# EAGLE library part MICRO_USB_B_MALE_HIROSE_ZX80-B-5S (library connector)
CONN PLUG MCR USB B PCB VERT
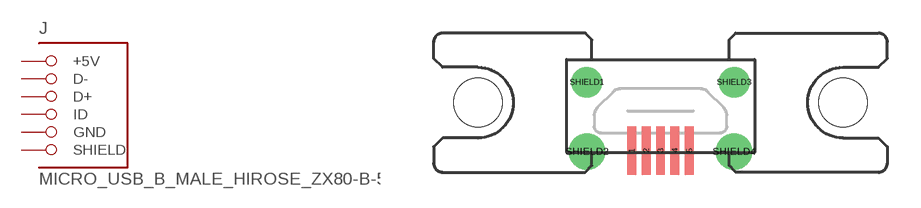
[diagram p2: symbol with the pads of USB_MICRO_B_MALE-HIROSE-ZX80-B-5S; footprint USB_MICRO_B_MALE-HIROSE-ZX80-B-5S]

Designator prefix J

## MICRO_USB_B_MALE_HIROSE_ZX80-B-5S (DIGIKEY: H11612-ND)  [USB_MICRO_B_MALE-HIROSE-ZX80-B-5S]
1  +5V
2  D-
3  D+
4  ID
5  GND
SHIELD1  SHIELD
SHIELD2  SHIELD
SHIELD3  SHIELD
SHIELD4  SHIELD

## Footprint USB_MICRO_B_MALE-HIROSE-ZX80-B-5S (pad centres in mm)
USB Male Micro B
smd 0.4 x 2.2: 1 -1.3,-1.8; 2 -0.65,-1.8; 3 0,-1.8; 4 0.65,-1.8; 5 1.3,-1.8
drill 0.762 pad 1.397: SHIELD1 -3.325,1.29; SHIELD3 3.325,1.29
drill 1.016 pad 1.651: SHIELD2 -3.325,-1.86; SHIELD4 3.325,-1.86
hole 2.2 at -8.252,0.37
hole 2.2 at 8.252,0.37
